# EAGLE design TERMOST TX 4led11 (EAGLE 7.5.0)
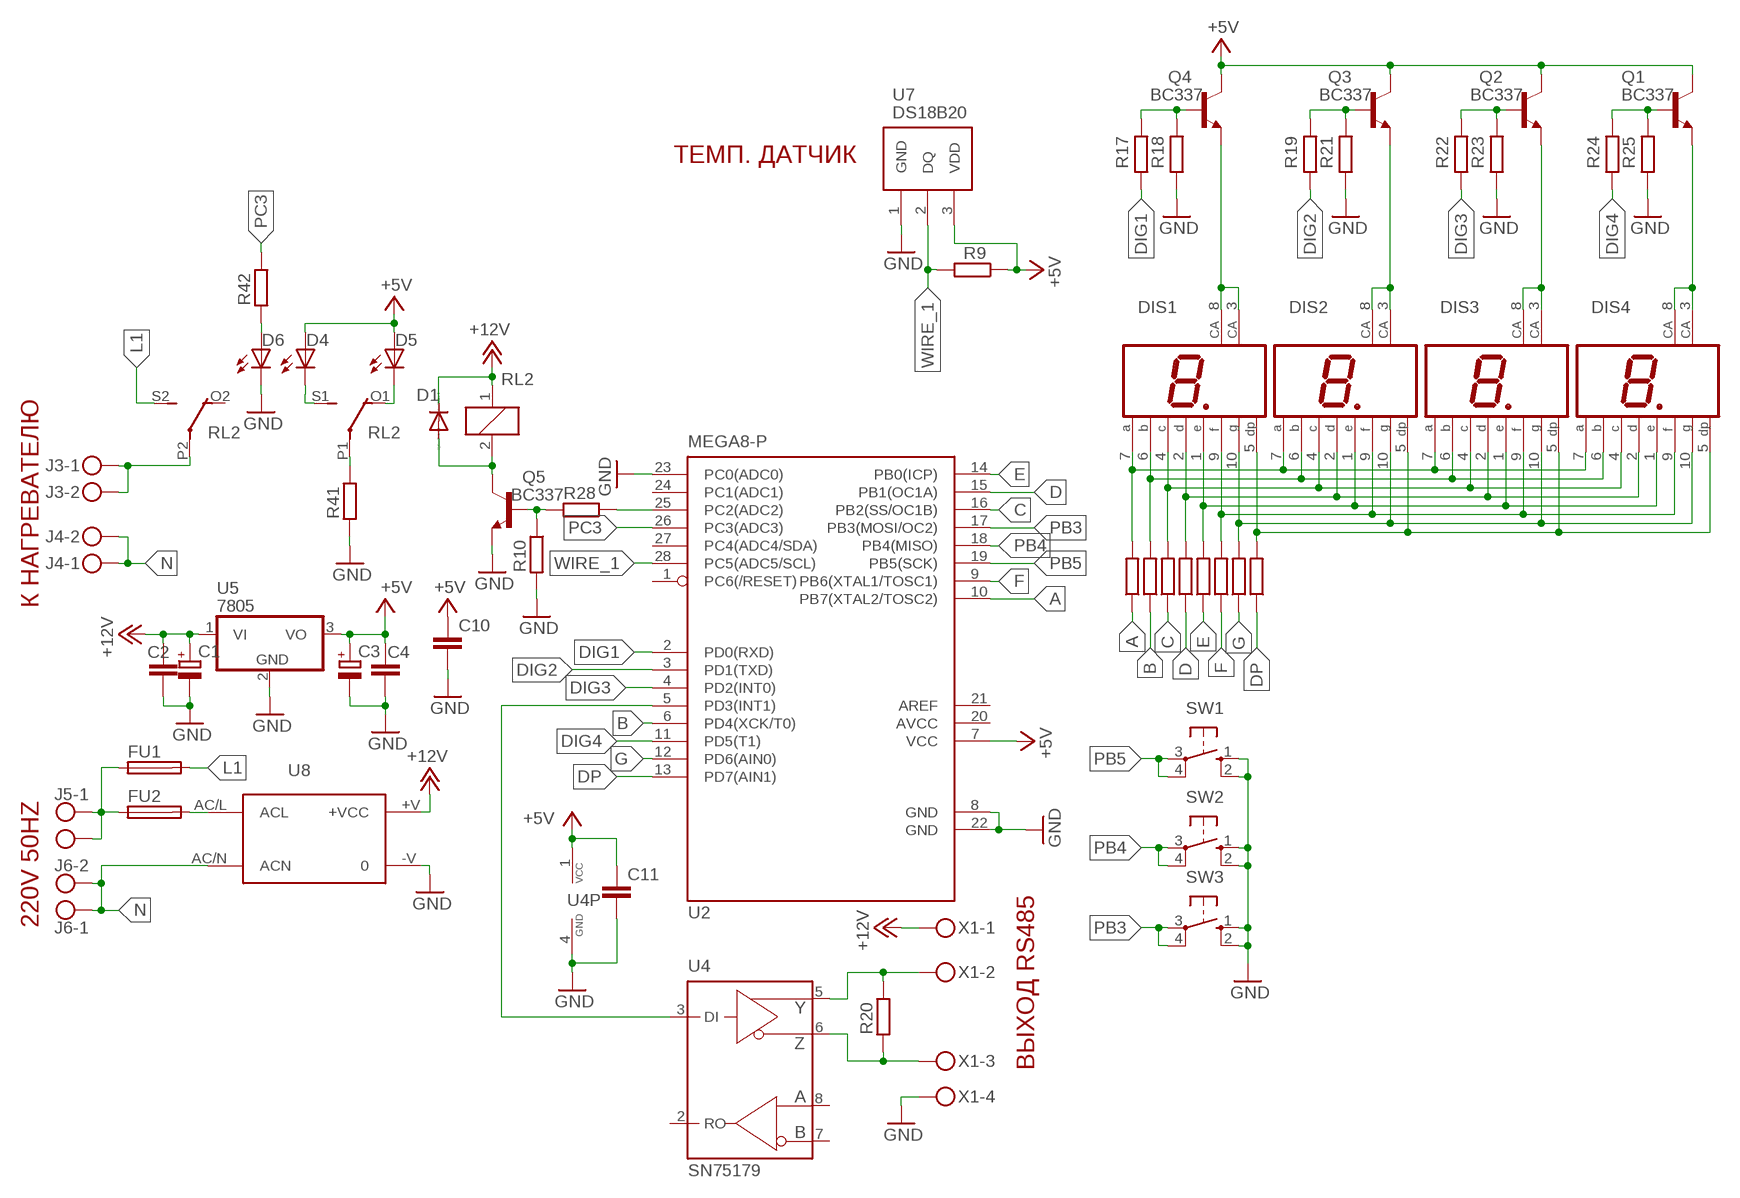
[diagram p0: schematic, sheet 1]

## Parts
C1  CPOL-EUE2.5-5  [E2,5-5]
C2  C-EUC1206  [C1206]
C3  CPOL-EUE2.5-5  [E2,5-5]
C4  C-EUC1206  [C1206]
C10  C-EUC1206  [C1206]
C11  C-EUC1206  [C1206]
D1  1N4004  [DO41-10]
D4  LED5MM  [LED5MM]
D5  LED5MM  [LED5MM]
D6  LED5MM  [LED5MM]
DIS1  HD-H101  [HDSP-M]
DIS2  HD-H101  [HDSP-M]
DIS3  HD-H101  [HDSP-M]
DIS4  HD-H101  [HDSP-M]
FU1  FUSEGSH15  [GSH15]
FU2  FUSEGSH15  [GSH15]
J3  MKDSN1,5/2-5,08  [MKDSN1,5/2-5,08]
J4  MKDSN1,5/2-5,08  [MKDSN1,5/2-5,08]
J5  MKDSN1,5/2-5,08  [MKDSN1,5/2-5,08]
J6  MKDSN1,5/2-5,08  [MKDSN1,5/2-5,08]
Q1  BC337  [TO92]
Q2  BC337  [TO92]
Q3  BC337  [TO92]
Q4  BC337  [TO92]
Q5  BC337  [TO92]
R1  R-EU_0204/7  [0204/7]
R2  R-EU_0204/7  [0204/7]
R3  R-EU_0204/7  [0204/7]
R4  R-EU_0204/7  [0204/7]
R5  R-EU_0204/7  [0204/7]
R6  R-EU_0204/7  [0204/7]
R7  R-EU_0204/7  [0204/7]
R8  R-EU_0204/7  [0204/7]
R9  R-EU_0204/7  [0204/7]
R10  R-EU_0204/7  [0204/7]
R17  R-EU_0204/7  [0204/7]
R18  R-EU_0204/7  [0204/7]
R19  R-EU_0204/7  [0204/7]
R20  R-EU_0204/7  [0204/7]
R21  R-EU_0204/7  [0204/7]
R22  R-EU_0204/7  [0204/7]
R23  R-EU_0204/7  [0204/7]
R24  R-EU_0204/7  [0204/7]
R25  R-EU_0204/7  [0204/7]
R28  R-EU_0204/7  [0204/7]
R41  R-EU_0204/7  [0204/7]
R42  R-EU_0204/7  [0204/7]
RL2  4052  [F4052]
SW1  10-XX  [B3F-10XX]
SW2  10-XX  [B3F-10XX]
SW3  10-XX  [B3F-10XX]
U2  MEGA8-P  [DIL28-3]
U4  SN75179  MAX488CPD  [DIL08]
U5  7805  7805T  [TO220H]
U7  DS18B20  [DS18B20]
U8  IRM10-12  [IRM10-12]
X1  MKDSN1,5/4-5,08  [MKDSN1,5/4-5,08]

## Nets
+5V: C3.+ C4.1 C10.1 C11.1 D4.A D5.A Q1.3(C) Q2.3(C) Q3.3(C) Q4.3(C) R9.1 U2.7(VCC) U4.1(VCC) U5.3(VO) U7.3(VDD)
+12V: C1.+ C2.1 D1.C RL2.1 U5.1(VI) U8.+V(+VCC) X1.1
A: R1.1 U2.10(PB7(XTAL2/TOSC2))
B: R2.1 U2.6(PD4(XCK/T0))
C: R3.1 U2.16(PB2(SS/OC1B))
D: R4.1 U2.15(PB1(OC1A))
DIG1: R17.1 U2.2(PD0(RXD))
DIG2: R19.1 U2.3(PD1(TXD))
DIG3: R22.1 U2.4(PD2(INT0))
DIG4: R24.1 U2.11(PD5(T1))
DP: R8.1 U2.13(PD7(AIN1))
E: R5.1 U2.14(PB0(ICP))
F: R6.1 U2.9(PB6(XTAL1/TOSC1))
G: R7.1 U2.12(PD6(AIN0))
GND: C1.- C2.2 C3.- C4.2 C10.2 C11.2 D6.K(C) Q5.1(E) R10.2 R18.1 R21.1 R23.1 R25.1 R41.2 SW1.1(S) SW1.2(S1) SW2.1(S) SW2.2(S1) SW3.1(S) SW3.2(S1) U2.8(GND) U2.22(GND) U2.23(PC0(ADC0)) U4.4(GND) U5.2(GND) U7.1(GND) U8.-V X1.4
L1: FU1.2 RL2.S2(3:S)
N: J4.1 J4.2 J6.1 J6.2 U8.AC/N(ACN)
N$1: DIS1.7(A) DIS2.7(A) DIS3.7(A) DIS4.7(A) R1.2
N$2: DIS1.6(B) DIS2.6(B) DIS3.6(B) DIS4.6(B) R2.2
N$3: DIS1.4(C) DIS2.4(C) DIS3.4(C) DIS4.4(C) R3.2
N$4: DIS1.2(D) DIS2.2(D) DIS3.2(D) DIS4.2(D) R4.2
N$5: DIS1.1(E) DIS2.1(E) DIS3.1(E) DIS4.1(E) R5.2
N$6: DIS1.9(F) DIS2.9(F) DIS3.9(F) DIS4.9(F) R6.2
N$7: DIS1.10(G) DIS2.10(G) DIS3.10(G) DIS4.10(G) R7.2
N$8: DIS1.5(DP) DIS2.5(DP) DIS3.5(DP) DIS4.5(DP) R8.2
N$9: DIS1.3(CA) DIS1.8(CA) Q4.1(E)
N$10: DIS2.3(CA) DIS2.8(CA) Q3.1(E)
N$11: Q4.2(B) R17.2 R18.2
N$12: Q3.2(B) R19.2 R21.2
N$13: DIS3.3(CA) DIS3.8(CA) Q2.1(E)
N$14: DIS4.3(CA) DIS4.8(CA) Q1.1(E)
N$15: Q2.2(B) R22.2 R23.2
N$16: Q1.2(B) R24.2 R25.2
N$17: R28.1 U2.25(PC2(ADC2))
N$18: Q5.2(B) R10.1 R28.2
N$20: D1.A Q5.3(C) RL2.2
N$21: D4.K(C) RL2.S1(2:S)
N$22: J3.1 J3.2 RL2.P2(3:P)
N$23: D5.K(C) RL2.O1(2:O)
N$24: D6.A R42.2
N$25: U2.5(PD3(INT1)) U4.3(DI)
N$26: R20.1 U4.5(Y) X1.2
N$27: R20.2 U4.6(Z) X1.3
N$28: FU1.1 FU2.1 J5.1 J5.2
N$29: FU2.2 U8.AC/L(ACL)
N$30: R41.1 RL2.P1(2:P)
PB3: SW3.3(P) SW3.4(P1) U2.17(PB3(MOSI/OC2))
PB4: SW2.3(P) SW2.4(P1) U2.18(PB4(MISO))
PB5: SW1.3(P) SW1.4(P1) U2.19(PB5(SCK))
PC3: R42.1 U2.26(PC3(ADC3))
WIRE_1: R9.2 U2.28(PC5(ADC5/SCL)) U7.2(DQ)
Unconnected: RL2.O2(3:O) U2.1(PC6(/RESET)) U2.21(AREF) U2.24(PC1(ADC1)) U2.27(PC4(ADC4/SDA)) U4.2(RO) U4.7(B) U4.8(A)

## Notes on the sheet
- ТЕМП. ДАТЧИК
- К НАГРЕВАТЕЛЮ
- 220V 50HZ
- ВЫХОД RS485

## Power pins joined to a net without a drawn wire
AVCC: U2.20(AVCC)

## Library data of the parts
C1 C3 = rcl:CPOL-EU: POLARIZED CAPACITOR, European symbol
C2 C4 C10 C11 = rcl:C-EU: CAPACITOR, European symbol
D1 = diode:1N4004: DIODE
D4-D6 = led:LED: LED
DIS1-DIS4 = display-hp:HD-H101: LED DISPLAY 1-character 7 segment, decimal point right; OC_FARNELL: unknown; OC_NEWARK: unknown
FU1 FU2 = fuse:FUSE: Fuse; OC_FARNELL: unknown; OC_NEWARK: unknown
J3-J6 = con-phoenix-508:MKDSN1,5/2-5,08: MKDSN 1,5/ 2-5,08 Printklemme
Q1-Q5 = transistor:BC337: NPN TRANSISTOR
R1-R10 R17-R25 R28 R41 R42 = rcl:R-EU_: RESISTOR, European symbol
RL2 = relay:4052: RELAY 2 x switch, Finder; OC_FARNELL: unknown; OC_NEWARK: unknown
SW1-SW3 = switch-omron:10-XX: OMRON SWITCH; MPN: B3F-1000; OC_FARNELL: 176432; OC_NEWARK: 36M3542
U2 = atmel:MEGA8-P: MICROCONTROLLER 8 Kbytes FLASH, 1 kbytes SRAM, 512 bytes EEPROM, USART, 4-channel 10 bit ADC, 2-channel 8 bit ADC Pin compatible with Atmega48, ATMega88, ATMega168 Source: avr.lbr; OC_FARNELL: unknown; OC_NEWARK: unknown
U4 = maxim:MAX488: RS485 TRANSEIVER Source: Data sheet; OC_FARNELL: unknown; OC_NEWARK: unknown
U5 = linear:78*: Positive VOLTAGE REGULATOR Source: http://cache.national.com/ds/LM/LM78L05.pdf http://www.fairchildsemi.com/ds/LM/LM7805.pdf
U7 = transistor:DS18B20
U8 = acdc:IRM10-12
X1 = con-phoenix-508:MKDSN1,5/4-5,08: MKDSN 1,5/ 4-5,08 Printklemme Nennstrom: 13,5 A Nennspannung: 250 V Rastermaß: 5,08 mm Polzahl: 4 Anschlussart: Schraubanschluss Montage: Löten Anschlussrichtung Leiter/Platine: 0 ° Artikelnummer: 1729144 Source: http://eshop.phoenixcontact.com .. 1729144.pdf

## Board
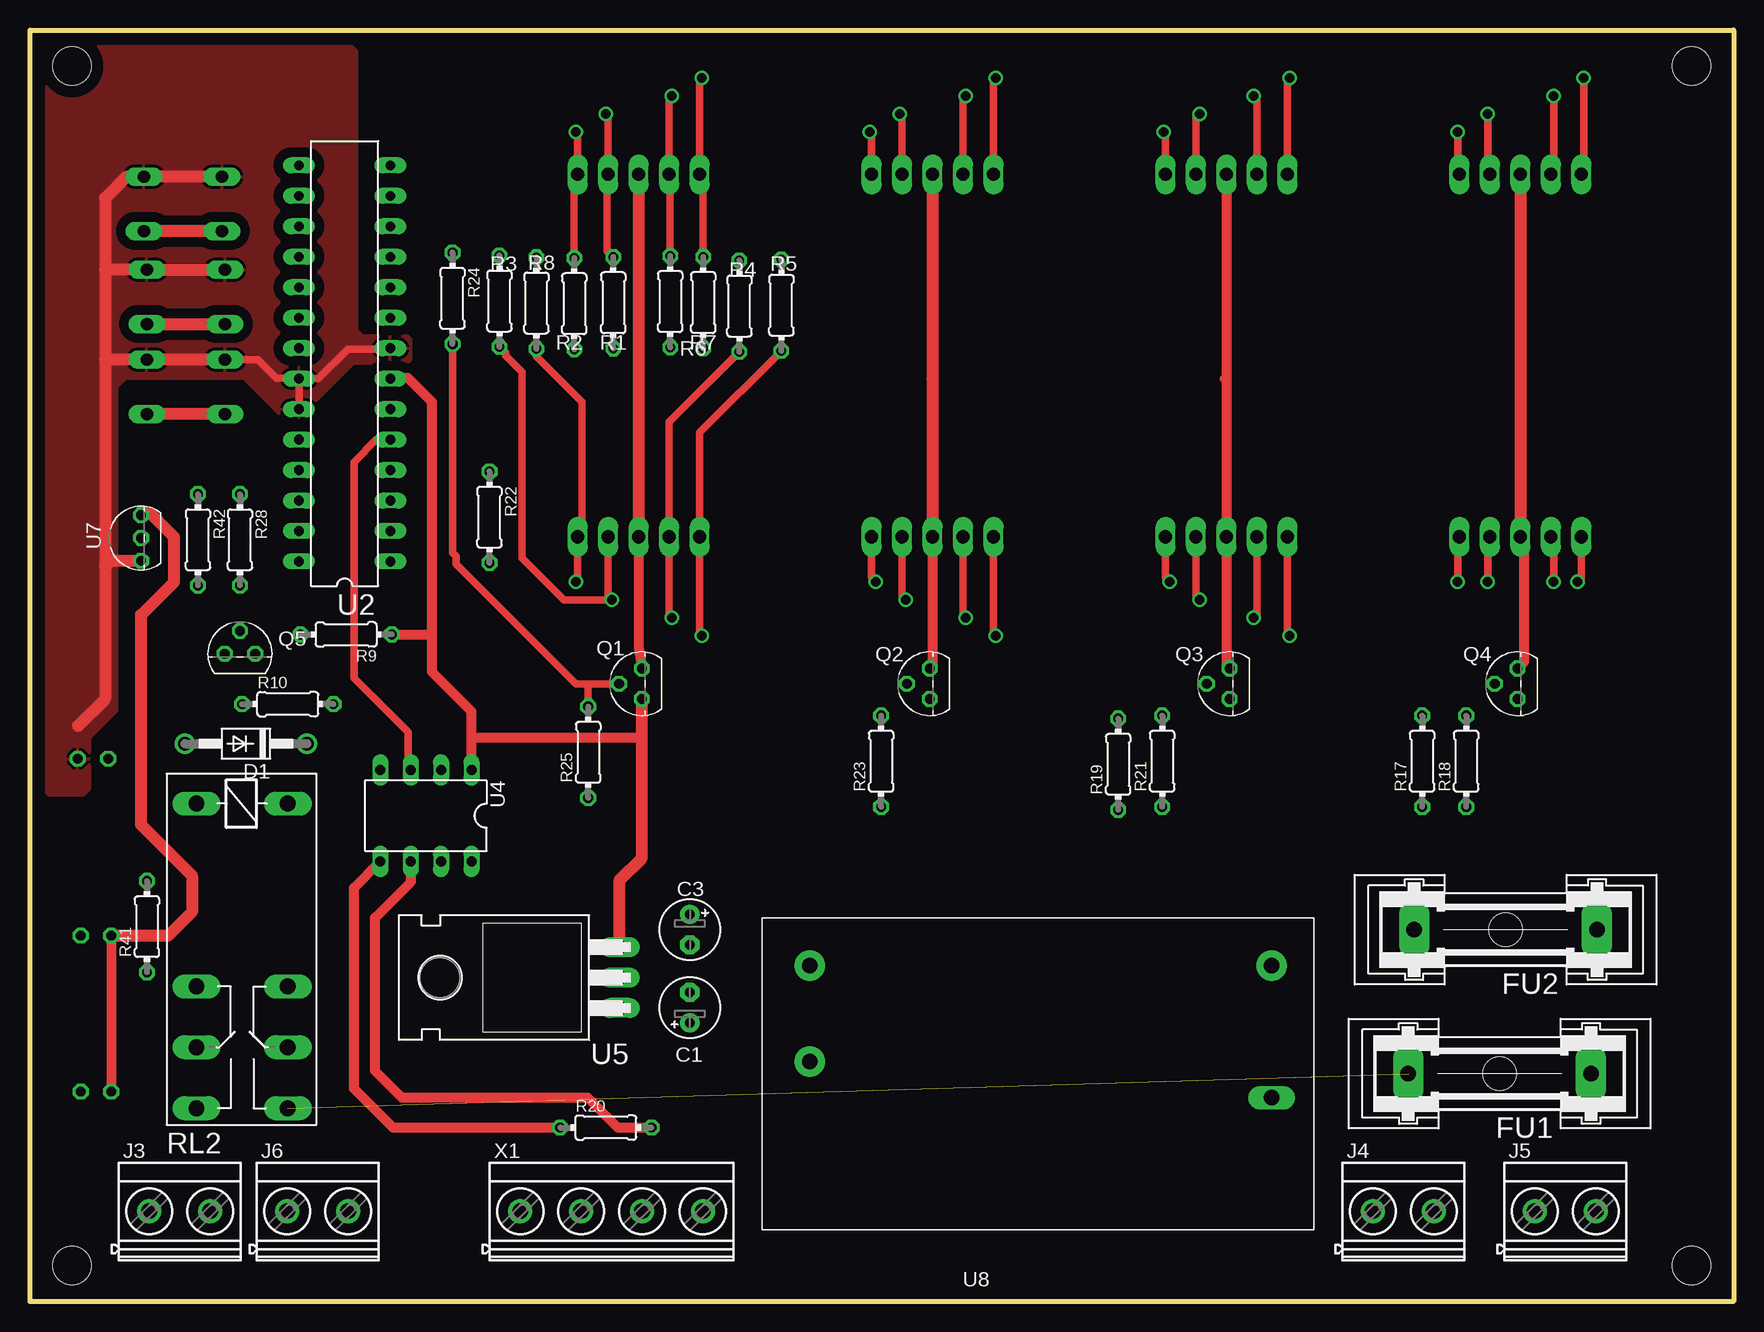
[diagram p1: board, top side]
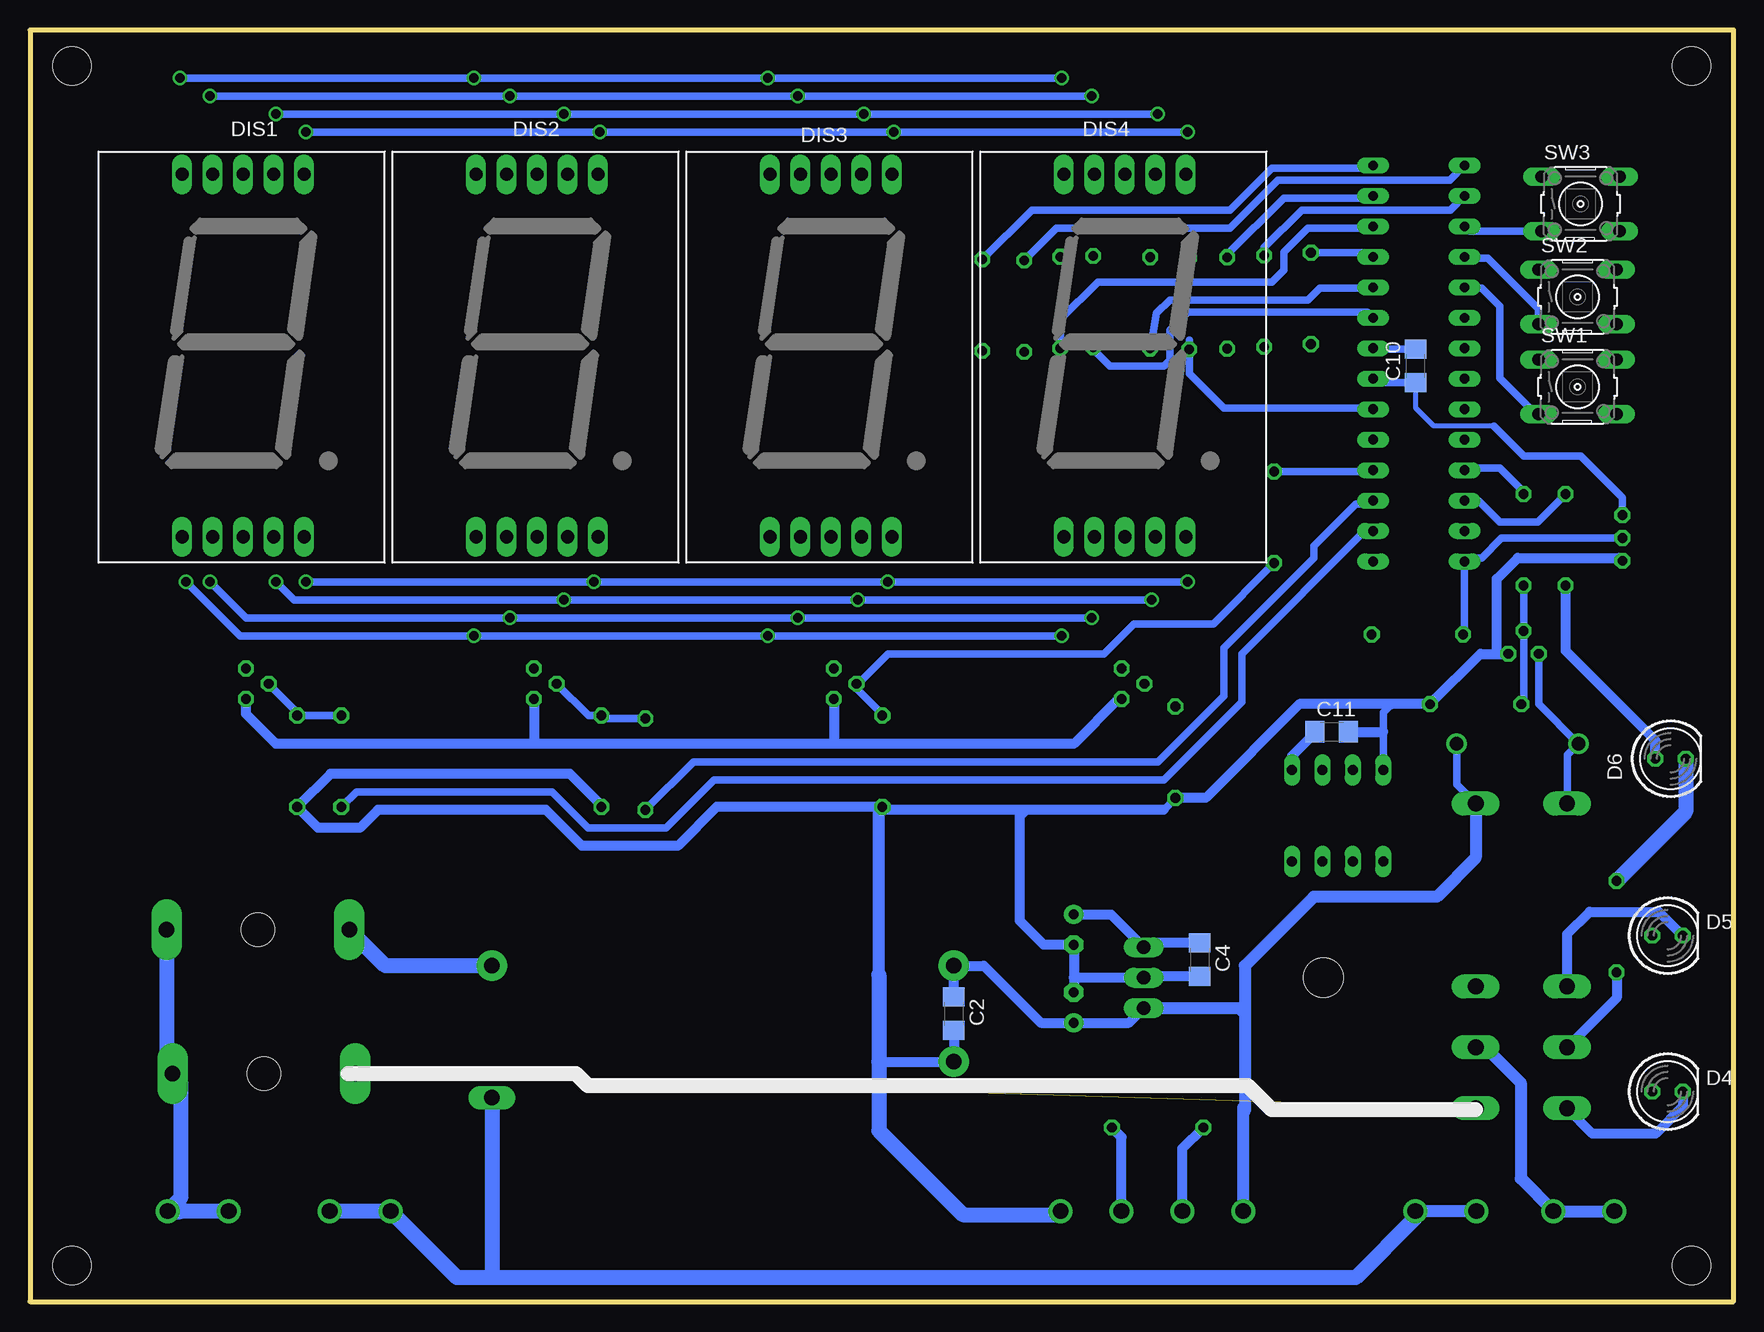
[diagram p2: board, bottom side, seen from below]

Size 142 x 106 mm. Coordinates in mm from the lower left corner, seen from the top.
Outline: 0,0 0,106 142,106 142,0 0,0
Copper layers (1*16): Top 0.035mm / dielectric 1.5mm / Bottom 0.035mm
Design rules "default": minimum track width 10mil, minimum drill 24mil, track to track 8mil, track to pad 8mil, pad to pad 8mil, via to via 8mil, smd to smd 8mil, copper to edge 40mil, drill to drill 8mil, minimum pad ring 10mil, minimum via ring 8mil, stop-mask expansion 4mil, vias tented up to drill 0mil, thermal gap 10mil
Holes 3.2 mm at 3.5,3 3.5,103 138.5,103 138.5,3

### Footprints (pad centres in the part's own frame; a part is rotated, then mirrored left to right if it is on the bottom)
E2,5-5 = drill 0.813 pad 1.6: + -1.27,0 | drill 0.813 pad 1.6 octagon: - 1.27,0
C1206 = smd 1.6 x 1.8: 1 -1.4,0; 2 1.4,0
DO41-10 = drill 1.118: A 5.08,0; C -5.08,0
LED5MM = drill 0.813 octagon: A -1.27,0; K 1.27,0
HDSP-M = drill 1.1 long: 1 -4.318,-16.256; 2 -1.778,-16.256; 3 0.762,-16.256; 4 3.302,-16.256; 5 5.842,-16.256; 6 5.842,13.97; 7 3.302,13.97; 8 0.762,13.97; 9 -1.778,13.97; 10 -4.318,13.97
GSH15 = drill 1.321 pad 2.54 long: 1 -7.62,0; 2 7.62,0 | hole 2.794: 0,0
MKDSN1,5/2-5,08 = drill 1.3 pad 2: 1 -2.561,0.025; 2 2.519,0.025
TO92 = drill 0.813 octagon: 1 1.27,0; 2 0,1.905; 3 -1.27,0
0204/7 = drill 0.813 octagon: 1 -3.81,0; 2 3.81,0
F4052 = drill 1.321 long: 1 -3.81,3.81; 2 -3.81,-3.81; O1 11.43,-3.81; O2 11.43,3.81; P1 16.51,-3.81; P2 16.51,3.81; S1 21.59,-3.81; S2 21.59,3.81
B3F-10XX = drill 1.016 long: 1 -3.251,2.261; 2 3.251,2.261; 3 -3.251,-2.261; 4 3.251,-2.261
DIL28-3 = drill 0.813 long: 1 -16.51,-3.81; 2 -13.97,-3.81; 3 -11.43,-3.81; 4 -8.89,-3.81; 5 -6.35,-3.81; 6 -3.81,-3.81; 7 -1.27,-3.81; 8 1.27,-3.81; 9 3.81,-3.81; 10 6.35,-3.81; 11 8.89,-3.81; 12 11.43,-3.81; 13 13.97,-3.81; 14 16.51,-3.81; 15 16.51,3.81; 16 13.97,3.81; 17 11.43,3.81; 18 8.89,3.81; 19 6.35,3.81; 20 3.81,3.81; 21 1.27,3.81; 22 -1.27,3.81; 23 -3.81,3.81; 24 -6.35,3.81; 25 -8.89,3.81; 26 -11.43,3.81; 27 -13.97,3.81; 28 -16.51,3.81
DIL08 = drill 0.813 long: 1 -3.81,-3.81; 2 -1.27,-3.81; 3 1.27,-3.81; 4 3.81,-3.81; 5 3.81,3.81; 6 1.27,3.81; 7 -1.27,3.81; 8 -3.81,3.81
TO220H = drill 1.118 long: 1 -2.54,-10.16; 2 0,-10.16; 3 2.54,-10.16 | hole 3.302: 0,4.826
DS18B20 = drill 0.813 octagon: 1 -3.175,0; 2 -1.27,0; 3 0.635,0
IRM10-12 = drill 1.3 pad 2.54: +V 38.5,0; -V 38.5,8; AC/L 0,0 | drill 1.3 long: AC/N 0,11
MKDSN1,5/4-5,08 = drill 1.3 pad 2: 1 -7.641,0.025; 2 -2.561,0.025; 3 2.519,0.025; 4 7.599,0.025

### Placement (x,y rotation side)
C1  55,24.5 90 top
C2  65,24 270 bottom
C3  55,31 270 top
C4  44.5,28.5 270 bottom
C10  26.5,78 90 bottom
C11  33.5,47.5 0 bottom
D1  18,46.5 180 top
D4  5.5,17.5 0 bottom
D5  5.5,30.5 0 bottom
D6  5.25,45.25 0 bottom
DIS1  125,80 0 bottom
DIS2  100.5,80 0 bottom
DIS3  76,80 0 bottom
DIS4  51.5,80 0 bottom
FU1  122.5,19 180 top
FU2  123,31 180 top
J3  12.5,7.5 0 top
J4  114.5,7.5 0 top
J5  128,7.5 0 top
J6  24,7.5 0 top
Q1  51,51.5 90 top
Q2  75,51.5 90 top
Q3  100,51.5 90 top
Q4  124,51.5 90 top
Q5  17.5,54 0 top
R1  48.62,83.26 90 top
R2  45.37,83.18 90 top
R3  39.13,83.4 270 top
R4  59.13,82.98 270 top
R5  62.63,83.06 270 top
R6  53.37,83.36 90 top
R7  56.12,83.28 90 top
R8  42.21,83.24 270 top
R9  26.35,55.61 180 top
R10  21.49,49.8 0 top
R17  116.05,45.04 90 top
R18  119.72,45.04 90 top
R19  90.71,44.79 90 top
R20  48,14.5 0 top
R21  94.38,45.04 90 top
R22  38.3,65.38 270 top
R23  70.95,45.04 90 top
R24  35.22,83.63 270 top
R25  46.53,45.79 90 top
R28  17.5,63.5 270 top
R41  9.75,31.25 90 top
R42  14,63.5 270 top
RL2  17.68,37.7 270 top
SW1  13,76.25 0 bottom
SW2  13,83.75 0 bottom
SW3  12.75,91.5 0 bottom
U2  26.23,78.2 90 top
U4  33,40.5 180 top
U5  39,27 90 top
U7  9.26,64.92 90 top
U8  103.5,28 180 top
X1  48.5,7.5 0 top

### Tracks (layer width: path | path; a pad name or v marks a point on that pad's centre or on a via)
+5V
  Top 0.813: Q1.3 51,50 | 33.5,55.5 33.5,52.5 36.81,49.19 36.81,47 | 33.5,55.5 33.5,75 31.5,77 30.11,77 U2.7 | U4.1 36.81,47 | R9.1 33.39,55.61 33.5,55.5 | 36.81,47 50.75,47 51,47.25 | D5.A D4.A
  Top 1.016: U7.3 9.46,65.75 10,65.75 12,63.75 12,60 9.25,57.25 9.25,39.75 13.5,35.5 13.5,32.5 11.5,30.5 D5.A | U5.3 49.16,35.16 51,37 51,47.25 Q1.3
  Bottom 0.406: 20,73 25,73 26.5,74.5 C10.1
  Bottom 0.61: C10.1 29.71,76.6 U2.7 | U7.3 9.26,67.01 12.75,70.5 17.5,70.5 20,73
  Bottom 0.813: Q1.3 51.27,50.23 55,46.5 75,46.5 | 75,46.5 100,46.5 | 100,46.5 121.5,46.5 124,49 Q4.3 | Q3.3 100,46.5 | Q2.3 75,46.5 | C11.1 34.9,47.41 36.81,45.5 U4.1 | C4.1 48.8,29.9 U5.3 51.89,32.27 C3.+
+12V
  Bottom 0.61: D1.C 23.08,43.1 RL2.1
  Bottom 0.813: U5.1 50.39,23.23 C1.+ 55.02,23.25 57.75,23.25 62.5,28 U8.+V C2.1
  Bottom 1.016: X1.1 40.86,15.75 | 40.86,15.75 40.86,16.16 | RL2.1 21.49,37.01 24.75,33.75 35,33.75 40.75,28 40.75,24 | 40.75,24 40.75,15.86 40.86,15.75 | U5.1 41.21,24.46 40.75,24
A
  Bottom 0.61: R1.1 48.12,82.38 47,83.5 35.5,83.5 34.5,84.5 30.09,84.5 U2.10
B
  Bottom 0.61: 45.37,80.13 R2.1 45.37,77.37 42.5,74.5 30.15,74.5 U2.6
C
  Bottom 0.61: R3.1 39.13,87.87 36,91 23.59,91 U2.16
D
  Bottom 0.61: U2.15 23.63,93.5 38,93.5 42,89.5 56.42,89.5 R4.1
DIG1
  Bottom 0.61: U2.2 30.77,64.23 41,54 41,50 47.5,43.5 85,43.5 89,39.5 95.5,39.5 98.5,42.5 114.78,42.5 R17.1
DIG2
  Bottom 0.61: U2.3 30.31,66.5 31.5,66.5 35,63 35,62 42.5,54.5 42.5,50.5 48,45 86.69,45 R19.1
DIG3
  Bottom 0.61: R22.1 30.16,69.19 U2.4
DIG4
  Bottom 0.61: R24.1 30.39,87.44 U2.11
DP
  Bottom 0.61: R8.1 42.21,87.29 37.5,92 30.21,92 U2.13
E
  Bottom 0.61: U2.14 30.25,94.5 38.5,94.5 42,91 58.5,91 R5.1
F
  Bottom 0.61: R6.1 53.37,79.37 52,78 47.5,78 47,78.5 47,81 45.5,82.5 30.53,82.5 U2.9
G
  Bottom 0.61: R7.1 56.12,81.88 53,85 38.5,85 37.5,86 37.5,87.5 35.5,89.5 30.17,89.5 U2.12
GND
  Top 0.61: SW1.1 18.99,78.51 20.5,77 22.35,77 U2.22 | U2.22 U2.23 | U2.22 24.03,76.93 C10.2 29.97,79.4 U2.8
  Top 1.016: SW3.2 SW3.1 8.01,93.76 6.25,92 6.25,86 | 6.25,86 6.26,86.01 SW2.2 SW2.1 | 6.25,86 6.25,78.5 | 6.25,78.5 6.25,61.25 | 6.25,61.25 6.25,50.25 3.98,47.98 | SW1.2 SW1.1 6.26,78.51 6.25,78.5 | U7.1 6.75,61.74 6.25,61.25
  Bottom 0.61: R25.1 47.5,41 | U4.4 29.19,47.5 29.19,49.11 28.5,49.8 | C10.2 29.97,79.4 U2.8
  Bottom 0.813: R21.1 94.38,41.38 97,44 116.95,44 R18.1 117.99,39.5 114.5,39.5 113,41 99,41 96,38 88,38 84.77,41.23 R23.1 70.72,41 59,41 | 47.5,41 59,41 | R25.1 46.51,42 44,42 36.2,49.8 28.5,49.8 R10.2 21.1,54 19.5,54 | C11.2 29.19,47.5 | U7.1 9.52,62 18,62 19.75,60.25 19.75,54.25 19.5,54 | C4.2 49.06,27.1 U5.2 55,27 | 55,27 C3.- 57.48,29.73 59.5,31.75 59.5,40.5 59,41 | 55,27 C1.- | 19.5,54 Q5.1 | C2.2 U8.-V 71.25,20
  Bottom 1.016: 71.25,27.25 71.25,40.93 R23.1
  Bottom 1.27: 71.25,27.25 71.25,20 71.25,14.25 64.25,7.25 56.37,7.25 X1.4 | D6.K 3.98,40.83 R41.2
  pour Top (isolate 0.813): 31.25,80.5 27.75,80.5 27.25,81 27.25,104.25 26.75,104.75 1.5,104.75 1.25,105 1.25,42.5 1.5,42.25 4.5,42.25 5,42.75 5,47 7.25,49.25 7.25,76.25 8,77 17.75,77 21,73.75 22.5,73.75 27,78.25 31.5,78.25 31.75,78.5 31.75,80.25 31.5,80.5
L1  (1 unrouted)
N
  Bottom 1.016: J6.1 J6.2
  Bottom 1.27: J6.2 26.52,6.98 31.5,2 103.5,2 | U8.AC/N 103.5,2 | 103.5,2 106.41,2 J4.1 J4.2
N$1  (via drill 0.8)
  Top 0.61: v48,99 48.2,98.8 DIS4.7 48.12,93.89 48.12,87.57 R1.2 | v121.5,99 121.5,94.17 DIS1.7 | DIS3.7 72.7,98.8 v72.5,99 | DIS2.7 97.2,98.7 v97.5,99
  Top 0.813: 121.62,93.89 DIS1.7
  Bottom 0.61: v48,99 v72.5,99 v97.5,99 v121.5,99
N$2  (via drill 0.8)
  Top 0.61: v45.5,97.5 45.66,97.34 DIS4.6 45.37,93.68 R2.2 | v119,97.5 119,94.13 DIS1.6 | DIS3.6 70.16,97.34 v70,97.5 | DIS2.6 94.66,97.34 v94.5,97.5
  Bottom 0.61: v45.5,97.5 v70,97.5 v94.5,97.5 v119,97.5
N$3  (via drill 0.8)
  Top 0.61: DIS4.4 48.2,58.8 v48.5,58.5 44.5,58.5 41,62 41,77.5 39.63,78.87 39.63,79.09 R3.2 | DIS1.4 121.5,63.55 v121.5,60 121.37,59.87 | DIS3.4 72.7,58.8 v73,58.5 | DIS2.4 97.2,58.8 v97.5,58.5
  Bottom 0.61: v48.5,58.5 v73,58.5 v97.5,58.5 120,58.5 v121.5,60
N$4  (via drill 0.8)
  Top 0.61: DIS2.2 102.28,57.28 v102,57 | v53.5,57 53.28,57.22 DIS4.2 53.28,73.32 R4.2 | DIS3.2 77.78,57.22 v78,57 | v127,60 127,63.52 DIS1.2
  Bottom 0.61: v53.5,57 v78,57 v102,57 124,57 v127,60
N$5  (via drill 0.8)
  Top 0.61: DIS2.1 104.82,55.68 v105,55.5 | v56,55.5 55.82,55.68 DIS4.1 55.82,72.44 R5.2 | DIS3.1 80.32,55.68 v80.5,55.5 | DIS1.1 129.32,60.32 v129,60
  Bottom 0.61: v56,55.5 v80.5,55.5 v105,55.5 124.5,55.5 v129,60
N$6  (via drill 0.8)
  Top 0.61: v53.5,100.5 53.28,100.28 DIS4.9 53.37,93.88 R6.2 | v127,100.5 127,94.19 DIS1.9 | DIS3.9 77.78,100.28 v78,100.5 | DIS2.9 102.28,100.22 v102,100.5
  Top 0.813: 126.87,93.88 DIS1.9
  Bottom 0.61: v53.5,100.5 v78,100.5 v102,100.5 v127,100.5
N$7  (via drill 0.8)
  Top 0.61: v56,102 55.82,101.82 DIS4.10 56.12,93.67 R7.2 | v129.5,102 129.5,94.15 DIS1.10 | DIS3.10 80.32,101.82 v80.5,102 | DIS2.10 104.82,101.82 v105,102
  Bottom 0.61: v56,102 v80.5,102 v105,102 v129.5,102
N$8  (via drill 0.8)
  Top 0.61: v45.5,60 45.66,60.16 DIS4.5 46,64.09 46,75 42.21,78.79 R8.2 | v119,60 119,63.59 DIS1.5 | DIS3.5 70.16,60.34 v70.5,60 | DIS2.5 94.66,60.34 v95,60
  Bottom 0.61: v45.5,60 v70.5,60 v95,60 v119,60 | DIS4.5 45.26,63.74
N$9
  Top 0.61: 124.5,63.48 DIS1.3 | 124.14,76.9 124.24,77
  Top 0.813: 124.5,63.48 124.5,53.27 Q4.1
  Top 1.016: DIS1.8 124.24,77 DIS1.3
N$10
  Top 0.813: DIS2.8 99.74,76.75 | 99.74,76.75 DIS2.3 99.74,53.03 Q3.1 | 99.59,76.9 99.74,76.75
N$11
  Bottom 0.61: R17.2 R18.2 119.72,49.12 Q4.2
  Bottom 0.813: 122.05,51.45 Q4.2
N$12
  Bottom 0.61: R19.2 94.13,48.6 R21.2 95.44,48.85 Q3.2
N$13
  Top 0.61: 75.25,64.24 75.24,64.25
  Top 0.813: 75.14,76.9 75.24,77 | DIS3.3 75.24,53.01 Q2.1
  Top 1.016: DIS3.8 75.24,77 75.24,64.25 DIS3.3
N$14
  Top 0.813: DIS4.3 50.74,54.53 Q1.1
  Top 1.016: DIS4.8 DIS4.3
N$15
  Bottom 0.61: R22.2 43.37,56.5 50,56.5 52.5,54 70.5,54 73,51.5 Q2.2 73,51.41 73,51 70.95,48.95 R23.2
N$16
  Top 0.61: R24.2 35.22,62.41 35.5,62.13 35.5,61.5 45.5,51.5 46.5,51.5 | Q1.2 46.5,51.5 | R25.2 46.53,51.47 46.5,51.5
N$17
  Bottom 0.61: R28.1 17.5,67.5 19.5,69.5 22.23,69.5 U2.25
N$18
  Bottom 0.61: R10.1 17.5,49.98 Q5.2 R28.2
N$20
  Bottom 0.61: Q5.3 16.23,49.81 D1.A 13.87,45.55 RL2.2
N$21
  Bottom 0.813: D4.K 4.23,16.27 6.5,14 11.76,14 RL2.S1
N$22
  Bottom 1.016: RL2.P2 20.69,21.19 17.75,18.25 17.75,10.26 J3.2 J3.1
N$23
  Bottom 0.813: RL2.O1 13.87,30.63 12,32.5 6.23,32.5 D5.K
N$24
  Bottom 0.813: R42.2 14,54.25 6.52,46.77 D6.A
N$25
  Top 0.61: U2.5 28.85,71.85 27,70 27,52 31.5,47.5 31.5,44.54 U4.3
N$26
  Top 0.813: R20.1 30.25,14.5 27,17.75 27,34.5 U4.5
  Bottom 0.813: X1.2 45.94,12.75 R20.1
N$27
  Top 0.813: R20.2 49,14.5 46.5,17 31,17 28.75,19.25 28.75,32 31.75,35 31.75,36.67 U4.6
  Bottom 0.813: X1.3 51.02,13.71 R20.2
N$28
  Bottom 1.27: FU2.1 130.62,19.63 130.75,19.5 130.62,19.5 FU1.1 129.44,18.32 129.44,8.61 J5.2 | J5.2 130.03,7.53 130,7.5 129.46,7.5 | J5.1 J5.2
N$29
  Bottom 1.27: U8.AC/L 112.38,28 FU2.2
N$30
  Bottom 0.813: R41.1 9.75,25.31 RL2.P1
PB3
  Top 1.016: SW3.3 SW3.4
  Bottom 0.61: SW3.3 22.03,89.24 U2.17
PB4
  Top 1.016: SW2.4 SW2.3
  Bottom 0.61: SW2.3 16.25,82.75 20.5,87 22.33,87 U2.18
PB5
  Top 1.016: SW1.3 SW1.4
  Bottom 0.61: SW1.3 16.49,73.99 19.5,77 19.5,83 21,84.5 22.37,84.5 U2.19
PC3
  Bottom 0.61: U2.26 21.27,66.77 19.5,65 16.31,65 R42.1
WIRE_1
  Bottom 0.61: R9.2 22.42,55.73 U2.28 22.11,62 21,62 19.35,63.65 U7.2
